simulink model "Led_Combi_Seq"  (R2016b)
settings: Solver=VariableStepAuto  StartTime=0.0  StopTime=inf  RelTol=1e-3
libraries: realtime_pacer_lib x1

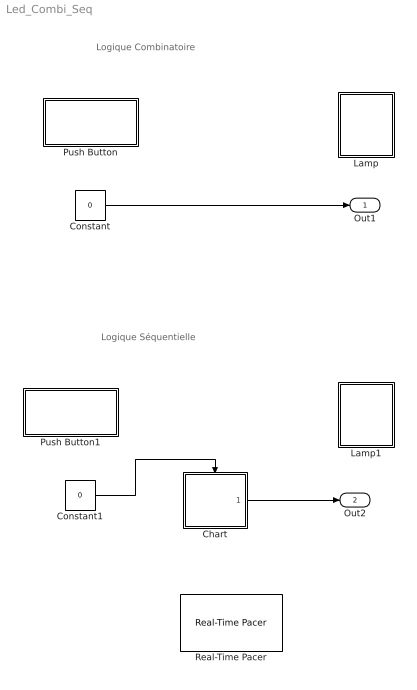
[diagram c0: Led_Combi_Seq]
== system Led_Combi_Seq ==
  note: Logique Combinatoire
  note: Logique Séquentielle
  Chart : Stateflow chart  TreatAsAtomicUnit=on
  Constant : Constant  Value=0
  Constant1 : Constant  Value=0
  Lamp : Subsystem  DialogController=hmiCreateDDGDialog  IsWebBlock=on
  Lamp1 : Subsystem  DialogController=hmiCreateDDGDialog  IsWebBlock=on
  Push Button : Subsystem  DialogController=hmiCreateDDGDialog  IsWebBlock=on
  Push Button1 : Subsystem  DialogController=hmiCreateDDGDialog  IsWebBlock=on
  Real-Time Pacer : realtime_pacer_lib/Real-Time Pacer  simTimePerRealTime=1
  Out1 : Outport
  Out2 : Outport  Port=2
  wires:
  Constant/1 -> Out1/1
  Constant1/1 -> Chart/Trigger
  Chart/1(S) -> Out2/1

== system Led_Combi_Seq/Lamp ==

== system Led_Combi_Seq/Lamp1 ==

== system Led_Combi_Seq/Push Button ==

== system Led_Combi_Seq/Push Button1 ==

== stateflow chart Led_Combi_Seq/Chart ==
  state OFF
    entry: S=0
  state ON
    entry: S=1
  (default) -> OFF
  OFF -> ON : a
  ON -> OFF : a
  data: S output
  events: input RISING_EDGE_EVENT
